PROGRAM MAIN
VAR
	hr : HRESULT; // 函数返回值
	fbCamera : FB_VN_SimpleCameraControl; // 视觉功能块
	eState : ETcVnCameraState; // TcVision 状态机
	ipImageIn : ITcVnImage; // 输入图像
	ipImageInDisp : ITcVnDisplayableImage; // 输入图像显示窗口
END_VAR

eState := fbCamera.GetState(); // 获取当前 TcVision 状态机
	CASE eState OF
		TCVN_CS_INITIAL,TCVN_CS_OPENING,TCVN_CS_OPENED,TCVN_CS_STARTACQUISITION:
			hr := fbCamera.StartAcquisition(); // 切换 TcVision 状态至工作模式
		TCVN_CS_ACQUIRING:
			hr := fbCamera.GetCurrentImage(ipImageIn); // 获取当前图片
			hr :=F_VN_TransformIntoDisplayableImage(ipImageIn , ipImageInDisp , hr );//转化为可显示图像
		TCVN_CS_ERROR:
			hr := fbCamera.Reset(); // TcVision 报错复位
END_CASE

END_PROGRAM
